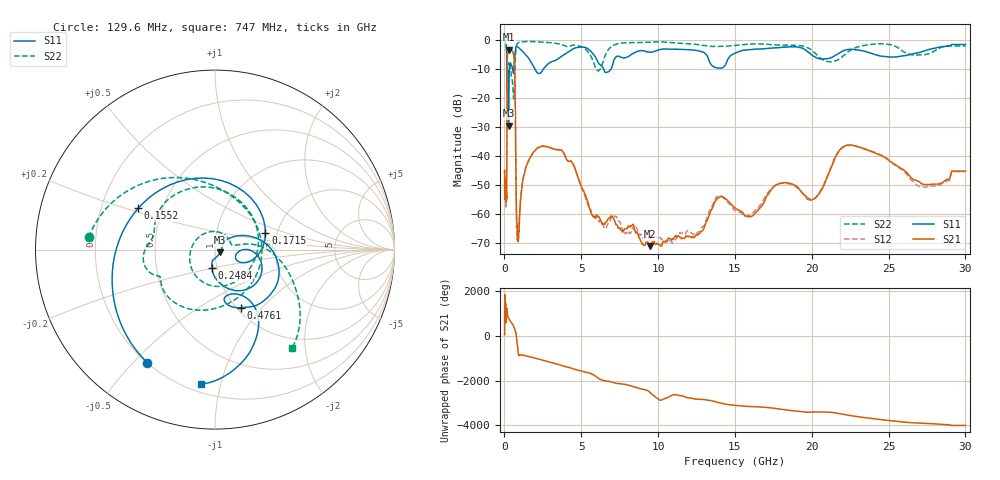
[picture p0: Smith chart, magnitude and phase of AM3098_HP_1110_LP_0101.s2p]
! Date/Time: Thu, Feb 28, 2019 8:46 AM
! Network Analyzer: Agilent Technologies E8364B Rev: A.07.50.67
! Sweep from 0.010 to 30.000 GHz, 1601 Points, Sweep Type: LOG
! Power Supply: 5.023 V, 0.002 A
# Hz S DB R 50
!freq MagS11 AngS11 MagS21 AngS21 MagS12 AngS12 MagS22 AngS22
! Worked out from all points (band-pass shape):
!   1601 points, 10 MHz to 30 GHz, reference 50 ohm
!   highest |S21| = -3.43 dB at 281.5 MHz (marker M1); lowest = -71.1 dB at 9.443 GHz (marker M2)
!   |S21| within 3 dB of the highest: 183.3 MHz to 624.2 MHz (440.8 MHz wide, 109 % of centre)
!   lowest |S11| = -29.6 dB at 263.8 MHz (marker M3), VSWR 1.07, Z = 53.1 - j1.5 ohm
!   |S11| at or under -10 dB: 170.1 MHz to 318.7 MHz (148.6 MHz wide, 60.8 % of centre); 1.975 GHz to 2.552 GHz (577.5 MHz wide, 25.5 % of centre); 6.445 GHz to 6.947 GHz (502.1 MHz wide, 7.5 % of centre)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
!   |S22| runs from -20.5 to -0.5 dB; largest |S21 - S12| = 0.0094
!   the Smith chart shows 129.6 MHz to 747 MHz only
!   S11 on the Smith chart (normalised r, x): 129.6 MHz: 0.20, -0.55; 155.2 MHz: 0.37, +0.22; 171.5 MHz: 1.74, +0.35; 248.4 MHz: 0.95, -0.20; 476.1 MHz: 1.05, -0.78; 747 MHz: 0.25, -0.87
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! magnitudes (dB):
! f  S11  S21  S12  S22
! 10 MHz  -0.4  -45.1  -45.7  -0.5
! 38.04 MHz  -0.3  -50.5  -51.3  -0.7
! 129.6 MHz  -2.7  -54.0  -51.5  -3.0
! 144.7 MHz  -4.3  -50.0  -51.4  -5.7
! 155.2 MHz  -6.3  -34.6  -34.3  -10.6
! 171.5 MHz  -10.6  -11.5  -11.5  -8.8
! 248.4 MHz  -19.7  -3.6  -3.6  -8.7
! 263.8 MHz  -29.6  -3.5  -3.4  -9.0
! 281.5 MHz  -18.2  -3.4  -3.4  -9.0
! 476.1 MHz  -9.0  -3.7  -3.7  -13.4
! 550.5 MHz  -11.0  -4.4  -4.3  -17.1
! 669.1 MHz  -6.1  -11.1  -11.1  -13.4
! 747 MHz  -2.5  -46.8  -46.9  -3.1
! 805.2 MHz  -2.3  -63.1  -68.2  -1.7
! 885.5 MHz  -2.6  -69.2  -66.2  -1.1
! 2.084 GHz  -11.1  -37.6  -37.7  -0.7
! 3.742 GHz  -5.6  -38.2  -38.1  -1.7
! 7.926 GHz  -6.2  -65.1  -66.8  -1.1
! 9.443 GHz  -4.3  -71.1  -67.9  -0.9
! 20 GHz  -5.3  -55.2  -55.0  -3.6
! 22.56 GHz  -3.3  -36.3  -36.4  -3.5
! 30 GHz  -1.7  -45.3  -45.5  -2.2
